FUNCTION_BLOCK FB_CSV_Access
VAR_INPUT
	
END_VAR
VAR_OUTPUT
	bError : BOOL := FALSE; 
	ipTcResult : I_TcMessage;
END_VAR
VAR

	sCmd : T_MaxString := '{ID};{Timestamp};{Name};{Velocity};{Temperature}'; 
	
	fbPLCDBCmd : FB_PLCDBCmdEvt(sNetID:= '', tTimeout := T#30S);
	
	para : ARRAY [0..4] OF ST_ExpParameter :=[
			(eParaType:= E_ExpParameterType.Int64, nParaSize := 8, sParaName := 'ID'),
			(eParaType:= E_ExpParameterType.DateTime, nParaSize := 4, sParaName := 'Timestamp'),
			(eParaType:= E_ExpParameterType.STRING_, nParaSize := 81, sParaName := 'Name'),
			(eParaType:= E_ExpParameterType.Double64, nParaSize := 8, sParaName := 'Velocity'),
			(eParaType:= E_ExpParameterType.Double64, nParaSize := 8, sParaName := 'Temperature')];

	fbPLCDBWrite: FB_PLCDBWriteEvt(sNetID:= '', tTimeout := T#30S);
	fbPLCDBRead : FB_PLCDBReadEvt(sNetID:= '', tTimeout := T#30S);			
	ColumnNames : ARRAY [0..4] OF STRING(50) := ['ID','Timestamp','Name','Velocity','Temperature'];  

END_VAR

METHOD ReadStruct : BOOL
VAR_INPUT
	hDBID : UDINT;
	
	pData : POINTER TO BYTE; //ARRAY[0..4] OF ST_CSVDataStruct;
	cbData: UDINT;
END_VAR
VAR	
END_VAR
ReadStruct := fbPLCDBRead.ReadStruct(
	hDBID:= hDBID, 
	sTableName:= 'CSV_Sample', 
	pColumnNames:= ADR(ColumnNames), 
	cbColumnNames:= SIZEOF(ColumnNames) , 
	sOrderByColumn:= 'ID', 
	eOrderType := E_OrderType.ASC, 
	nStartIndex:=  0, 
	nRecordCount:= 5, 
	pData:= pData, 
	cbData:= cbData);

IF ReadStruct THEN
	IF fbPLCDBRead.bError THEN
		ipTcResult := fbPLCDBRead.ipTcResult;
		bError:= TRUE;
	END_IF
END_IF
END_METHOD

METHOD Write : BOOL
VAR_INPUT
	hDBID : UDINT;
	InputData: ST_CSVDataStruct;	
END_VAR
Write := fbPLCDBCmd.Execute(
	hDBID:= hDBID, 
	pExpression:= ADR(sCmd), 
	cbExpression:= SIZEOF(sCmd), 
	pData:= ADR(InputData), 
	cbData:= SIZEOF(InputData) , 
	pParameter:=  ADR(para), 
	cbParameter:=SIZEOF(para));
	
IF Write THEN
	IF fbPLCDBCmd.bError THEN
		ipTcResult := fbPLCDBCmd.ipTcResult;
		bError:= TRUE;
	END_IF
END_IF
END_METHOD

METHOD WriteStruct : BOOL
VAR_INPUT
	hDBID : UDINT;
	Data : ST_CSVDataStruct; 
END_VAR
VAR
	
END_VAR
WriteStruct := fbPLCDBWrite.WriteStruct(
	hDBID:= hDBID, 
	sTableName:= 'CSV_Sample', 
	pRecord:= ADR(Data), 
	cbRecord:= SIZEOF(Data), 
	pColumnNames:= ADR(ColumnNames), 
	cbColumnNames:= SIZEOF(ColumnNames) );

IF WriteStruct THEN
	IF fbPLCDBWrite.bError THEN
		ipTcResult := fbPLCDBWrite.ipTcResult;
		bError:= TRUE;
	END_IF
END_IF
END_METHOD

END_FUNCTION_BLOCK
